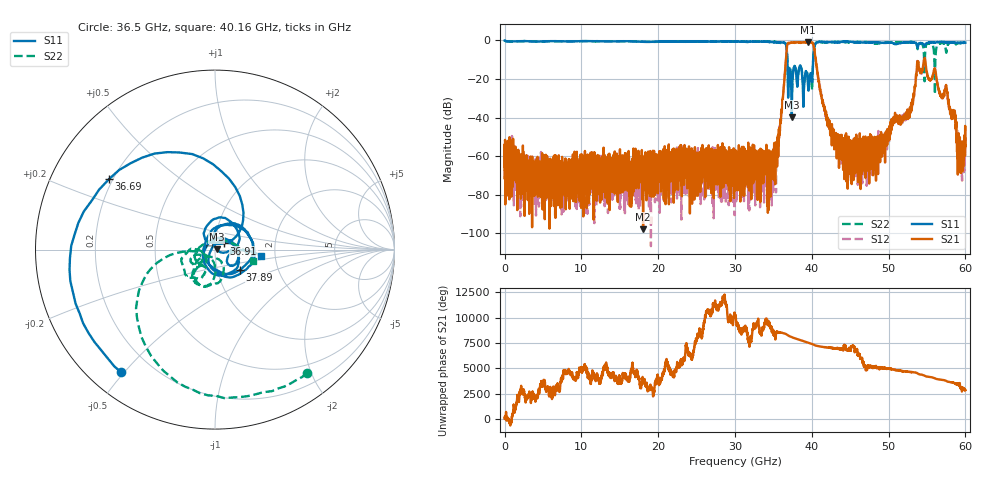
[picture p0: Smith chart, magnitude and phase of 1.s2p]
! 2/14/2023 10:19:31 AM
! C:\USERS\VECTORSTARUSER\DESKTOP\_XLC\ZBF6-C38.5-3G-1354\1.S2P
! CHANNEL.1
! TR.MEASUREMENT
! CORRECTED.DATA
! RF.CORRECTION: FULL.TWO.PORT.CAL.PORT.1.2
! AVERAGING.OFF
! IF.BANDWIDTH: 100KHZ
! SWEEPTYPE:  FREQ.SWEEP(Linear)
! Reference Plane Port Info
! PORT:  PORT1  PORT2
! DISTANCE:  0  m  0  m
! TIME:  0  s  0  s
! PHASE.OFFSET:  0 °  0 °
! LOSS:  0  dB  0  dB
! REF.LOSS:  0  dB  0  dB
! REF.FREQ:  0  Hz  0  Hz
! Power Info
! POWER:  -10  dBm  -10  dBm
! EFF.POWER:  -10  dBm  -10  dBm
! SOURCE.ATTEN:  0  dB  0  dB
! TEST.ATTEN:  0  dB  0  dB
# GHZ S RI R 50.0
! FREQ.GHZ  S11RE  S11IM  S21RE  S21IM  S12RE  S12IM  S22RE  S22IM
!; PortSelection: Port_12
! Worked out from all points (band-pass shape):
!   6001 points, 10 MHz to 60.01 GHz, reference 50 ohm
!   highest |S21| = -0.90 dB at 39.54 GHz (marker M1); lowest = -98.1 dB at 18.04 GHz (marker M2)
!   |S21| within 3 dB of the highest: 36.76 GHz to 40.29 GHz (3.529 GHz wide, 9.16 % of centre)
!   lowest |S11| = -39.9 dB at 37.4 GHz (marker M3), VSWR 1.02, Z = 51 + j0.0811 ohm
!   |S11| at or under -10 dB: 36.82 GHz to 40.18 GHz (3.36 GHz wide, 8.73 % of centre)
!   |S22| runs from -27.9 to 0.0 dB; largest |S21 - S12| = 0.11
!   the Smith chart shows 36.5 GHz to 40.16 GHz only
!   S11 on the Smith chart (normalised r, x): 36.5 GHz: 0.09, -0.49; 36.69 GHz: 0.19, +0.29; 36.91 GHz: 1.10, +0.08; 37.89 GHz: 1.28, -0.30; 40.16 GHz: 1.68, -0.13
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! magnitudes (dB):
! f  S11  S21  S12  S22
! 10 MHz  -0.1  -65.6  -67.7  0.0
! 10.01 GHz  -0.4  -66.1  -73.6  -0.4
! 18.04 GHz  -0.8  -98.1  -63.4  -0.7
! 20.01 GHz  -0.6  -65.5  -63.2  -0.7
! 30.01 GHz  -0.6  -59.7  -69.7  -0.5
! 35.05 GHz  -1.0  -61.9  -74.5  -0.6
! 36.5 GHz  -1.3  -16.6  -17.9  -1.3
! 36.69 GHz  -3.0  -7.2  -7.4  -2.5
! 36.91 GHz  -24.3  -1.4  -1.4  -23.3
! 37.4 GHz  -39.9  -1.1  -1.1  -26.6
! 37.89 GHz  -14.9  -1.2  -1.2  -14.3
! 39.54 GHz  -24.6  -0.9  -1.0  -20.1
! 40.01 GHz  -20.7  -1.1  -1.0  -23.4
! 40.16 GHz  -11.8  -1.9  -1.4  -13.2
! 41.94 GHz  -0.9  -39.0  -39.9  -1.0
! 43.85 GHz  -0.8  -53.3  -56.5  -0.7
! 50.01 GHz  -1.2  -47.8  -49.0  -1.0
! 52.77 GHz  -1.1  -36.2  -37.2  -0.9
! 54.66 GHz  -2.8  -9.3  -9.7  -14.5
! 57.52 GHz  -1.0  -23.9  -25.0  -6.4
! 59.14 GHz  -1.3  -57.3  -57.2  -1.4
! 60.01 GHz  -1.2  -54.8  -55.6  -1.6
